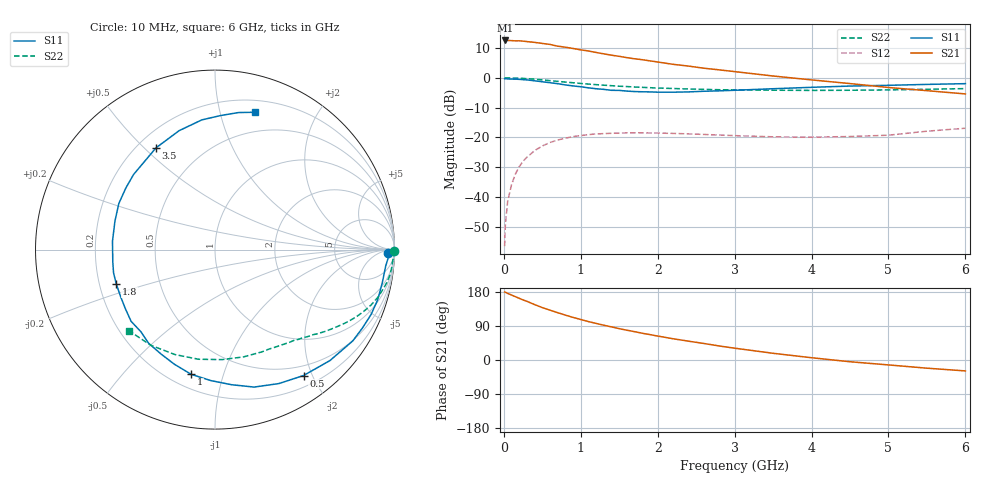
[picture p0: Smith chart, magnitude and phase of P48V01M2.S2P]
! SIEMENS Small Signal Semiconductors
! BFP182
! Si NPN RF Bipolar Junction Transistor in SOT143
! VCE = 8 V  IC = 1.2 mA
! Common Emitter S-Parameters:  March  1996
# GHz  S  MA  R  50
!  f  S11  S21  S12  S22
! GHz  MAG  ANG  MAG  ANG  MAG  ANG  MAG  ANG
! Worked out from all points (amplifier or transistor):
!   36 points, 10 MHz to 6 GHz, reference 50 ohm
!   highest |S21| = 12.5 dB at 20 MHz (marker M1)
!   |S21| within 3 dB of that: start of sweep to 966.6 MHz
!   unconditionally stable (mu >= 1): 2.576 GHz to end of sweep
!   at 250 MHz: K = 0.11, MSG = 20.1 dB, |S12| = -28.0 dB
!   at 1.4 GHz: K = 0.57, MSG = 13.1 dB, |S12| = -18.6 dB
!   at 6 GHz: K = 1.05, MAG = 4.4 dB, |S12| = -16.9 dB
!   S11 on the Smith chart (normalised r, x): 10 MHz: 42, -22; 500 MHz: 0.35, -1.87; 1 GHz: 0.28, -0.79; 1.8 GHz: 0.27, -0.16; 3.5 GHz: 0.27, +0.54; 6 GHz: 0.31, +1.29
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0.01  0.9634 -1.1  4.222 179.4  0.0015 92.2  0.9966 -0.4
0.02  0.9669 -2.5  4.226 178.9  0.0035 92.6  0.9959 -0.9
0.05  0.9552 -5.6  4.226 175.7  0.0085 89.9  0.9962 -2.1
0.1  0.9503 -11.2  4.201 171.4  0.0161 81.3  0.9907 -4.3
0.15  0.9486 -17.1  4.159 167.1  0.0243 79.4  0.9891 -6.3
0.2  0.9418 -22.6  4.172 162.8  0.0322 76.1  0.9839 -8.4
0.3  0.921 -33.5  4.047 154.9  0.0466 69.5  0.9664 -12.4
0.4  0.8901 -44.0  3.923 146.2  0.0601 63.2  0.9473 -16.1
0.5  0.8576 -54.9  3.77 138.3  0.0718 56.9  0.9224 -19.6
0.6  0.8269 -64.5  3.623 131.5  0.0822 51.4  0.8962 -22.7
0.8  0.7585 -83.0  3.258 118.4  0.0969 41.7  0.847 -28.0
1  0.7075 -100.8  2.94 106.8  0.1072 33.8  0.8038 -32.3
1.1  0.6777 -109.5  2.814 101.3  0.1115 30.3  0.784 -34.4
1.3  0.6394 -125.4  2.52 91.8  0.1159 23.9  0.7511 -38.0
1.5  0.6149 -139.5  2.289 82.7  0.118 19.0  0.7219 -41.1
1.8  0.5824 -160.8  2.009 70.6  0.1196 13.3  0.691 -45.5
2.2  0.5731 175.3  1.682 56.1  0.1167 7.2  0.6614 -51.6
2.8  0.604 145.2  1.358 37.0  0.1096 3.1  0.6306 -61.5
3.5  0.6553 120.1  1.071 17.7  0.1023 3.0  0.6185 -75.1
4.5  0.7264 95.8  0.8 -4.6  0.1035 10.1  0.6177 -98.5
5.5  0.7746 80.3  0.608 -21.6  0.1271 16.5  0.6421 -123.9
6  0.7969 73.8  0.536 -28.8  0.1426 15.2  0.6584 -136.5
